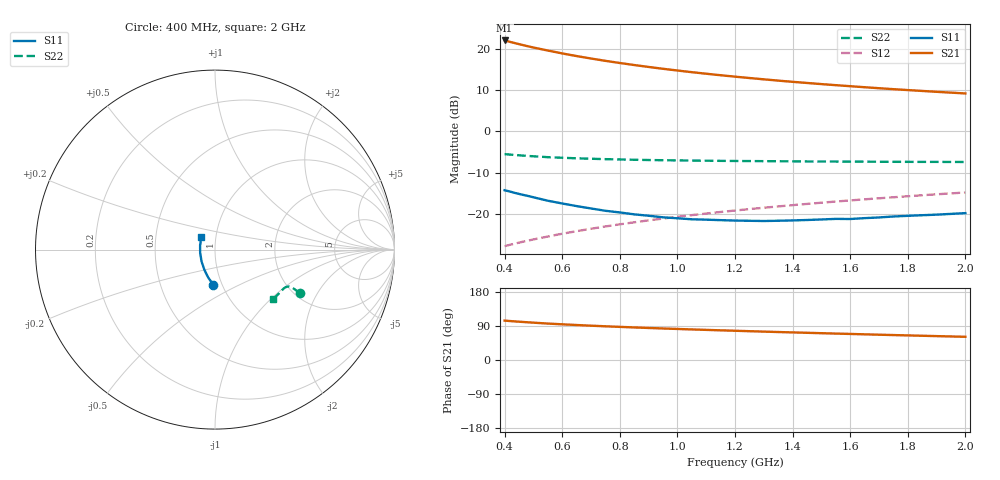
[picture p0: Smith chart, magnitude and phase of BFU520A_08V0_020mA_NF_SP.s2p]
! Filename:  P:\Prog\Test\Noise\ATS_data\Testdata_Net\06 Compressed Noise after Statistics\BFU520A_APG2013_30_A05_08p0V_020mA_NF_CM01_D.sf
! Date/Time: Wed 24/Apr/2013 20:06:20
! BFU520A_APG2013_30_A05_08p0V_1to20mA_NF_CM01_Bias8_R.sf
! Noise Parameter Data File
! BFU520A_APG2013_30_A05_08p0V_1to20mA_NF_CM01
! Date/time: Thu Apr 11 09:33:54 2013
! VAR V_out= 8.000000
! VAR I_out= 19.995000
! VAR V_in= 0.826600
! VAR I_in= 0.216650
! Device data file deembeded for feedlines and parallel
! Original file: \06 Compressed Noise after Statistics\BFU520A_APG2013_30_A05_08p0V_020mA_NF_CM01_R.sf
! Feed-files: PR017V01_150413_Feed1.s2p, PR017V01_150413_Feed2.s2p
! Parallel-file: PR017V01_150413_Par.s2p
# MHz S MA R 50
!  Freq-MHz  S11-mag  S11-arg  S21-mag  S21-arg  S12-mag  S12-arg  S22-mag  S22-arg
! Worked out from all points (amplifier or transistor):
!   37 points, 400 MHz to 2 GHz, reference 50 ohm
!   highest |S21| = 22.0 dB at 400 MHz (marker M1)
!   |S21| within 3 dB of that: start of sweep to 590.4 MHz
!   unconditionally stable (mu >= 1): 986.5 MHz to 1.827 GHz
!   at 500 MHz: K = 0.93, MSG = 23.2 dB, |S12| = -26.1 dB
!   at 1.1 GHz: K = 1.00, MAG = 16.5 dB, |S12| = -19.8 dB
!   at 2 GHz: K = 1.00, MSG = 12.0 dB, |S12| = -14.8 dB
!   lowest NFmin = 1.15 dB at 420 MHz
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400  0.1948 -92.6  12.58 104.0  0.04104 73.9  0.5322 -27.0
420  0.1872 -95.0  12.06 102.7  0.04275 74.1  0.5244 -26.9
440  0.1792 -97.2  11.58 101.6  0.04441 74.2  0.5178 -26.8
460  0.1724 -99.2  11.13 100.5  0.04613 74.4  0.5118 -26.8
480  0.1664 -101.5  10.72 99.5  0.04779 74.5  0.5055 -26.7
500  0.16 -103.7  10.34 98.5  0.04949 74.7  0.5007 -26.6
550  0.1454 -108.8  9.504 96.2  0.0537 75.0  0.4886 -26.4
600  0.1346 -113.7  8.768 94.2  0.058 75.2  0.4806 -26.3
650  0.1252 -118.5  8.149 92.3  0.06229 75.3  0.4733 -26.4
700  0.1172 -123.3  7.609 90.5  0.06664 75.5  0.4676 -26.4
750  0.1099 -128.2  7.133 88.9  0.071 75.5  0.4625 -26.5
800  0.1049 -133.2  6.719 87.4  0.07535 75.6  0.4583 -26.7
850  0.09946 -138.5  6.349 85.9  0.07974 75.5  0.4545 -27.0
950  0.09158 -148.0  5.718 83.2  0.08851 75.4  0.4489 -27.6
1050  0.08673 -157.7  5.204 80.7  0.09733 75.3  0.4444 -28.4
1150  0.08467 -167.6  4.779 78.3  0.1062 75.0  0.4408 -29.3
1200  0.08371 -171.4  4.594 77.2  0.1107 74.8  0.4394 -29.8
1350  0.08325 175.4  4.114 73.8  0.124 74.2  0.4362 -31.4
1500  0.08628 163.9  3.734 70.8  0.1375 73.5  0.4328 -33.2
1650  0.08956 154.3  3.423 67.8  0.1512 72.6  0.4312 -35.3
1750  0.09374 148.8  3.242 65.8  0.1601 72.0  0.4292 -36.6
2000  0.1029 137.1  2.878 61.2  0.1829 70.5  0.4271 -40.4
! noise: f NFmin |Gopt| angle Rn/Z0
400  1.185  0.1973  -164.5  0.1023
460  1.19  0.2094  -165.3  0.0908
600  1.302  0.1727  -151.5  0.123
800  1.22  0.2197  -152.2  0.1016
1000  1.256  0.2437  -146.8  0.1007
1200  1.3  0.2452  -140.5  0.1106
1400  1.348  0.2649  -135.5  0.0993
1600  1.335  0.2827  -129.9  0.1159
1800  1.319  0.3053  -125.7  0.1213
2000  1.36  0.3092  -121.2  0.1332
